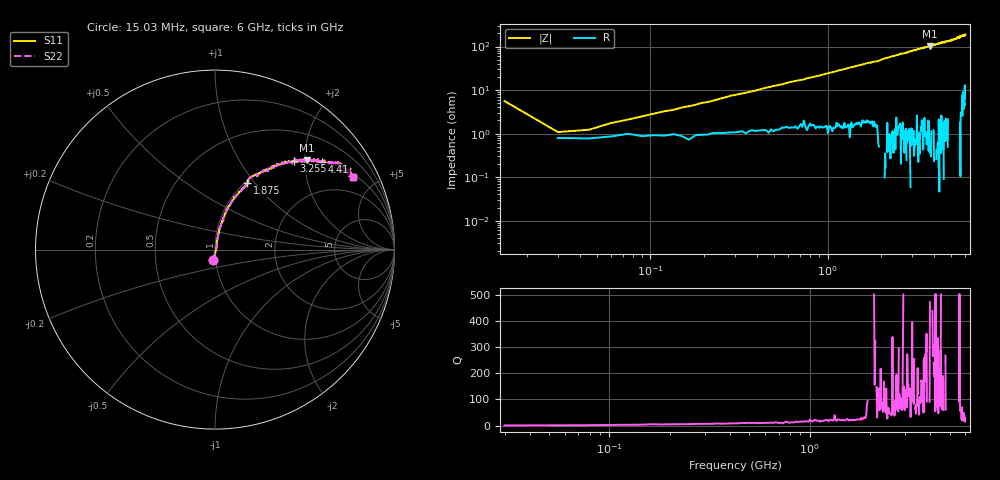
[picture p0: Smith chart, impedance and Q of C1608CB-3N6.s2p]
!	Network	Analyzer	HP8753E.07.74:	Oct	30	2002	Serial	No.	JP38451487
!	Hewlett-Packard
!	27	Aug	2009	15:19:33
!	Frequency	S11	S21	S12	S22
#	HZ	S	RI	R	50
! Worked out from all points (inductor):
!   400 points, 15.03 MHz to 6 GHz, reference 50 ohm
!   read as one part in series: L = 3.94 nH near 45.03 MHz
!   highest Q = 260 at 3.78 GHz (marker M1), where L = 4.32 nH
!   S11 on the Smith chart (normalised r, x): 15.03 MHz: 0.98, -0.11; 1.875 GHz: 1.03, +0.91; 3.255 GHz: 1.00, +1.77; 4.41 GHz: 1.01, +2.44; 6 GHz: 1.13, +3.73
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1.502992e7  -0.00853 -0.0557  1.01 0.0557  1.01 0.0557  -0.00853 -0.0557
3.002985e7  0.00785 0.00728  0.992 -0.00728  0.992 -0.00728  0.00785 0.00728
4.502978e7  0.00755 0.00938  0.992 -0.00938  0.992 -0.00938  0.00755 0.00938
6.00297e7  0.00855 0.015  0.991 -0.015  0.991 -0.015  0.00855 0.015
7.502962e7  0.0103 0.0182  0.99 -0.0182  0.99 -0.0182  0.0103 0.0182
1.200294e8  0.00975 0.0308  0.99 -0.0308  0.99 -0.0308  0.00975 0.0308
2.850286e8  0.0157 0.072  0.984 -0.072  0.984 -0.072  0.0157 0.072
6.150269e8  0.0354 0.145  0.965 -0.145  0.965 -0.145  0.0354 0.145
1.020025e9  0.0694 0.226  0.931 -0.226  0.931 -0.226  0.0694 0.226
1.875021e9  0.18 0.369  0.82 -0.369  0.82 -0.369  0.18 0.369
2.01002e9  0.198 0.401  0.802 -0.401  0.802 -0.401  0.198 0.401
3.015015e9  0.391 0.491  0.609 -0.491  0.609 -0.491  0.391 0.491
3.255014e9  0.439 0.495  0.561 -0.495  0.561 -0.495  0.439 0.495
3.780011e9  0.513 0.498  0.487 -0.498  0.487 -0.498  0.513 0.498
4.00501e9  0.551 0.504  0.449 -0.504  0.449 -0.504  0.551 0.504
4.410008e9  0.598 0.488  0.402 -0.488  0.402 -0.488  0.598 0.488
5.010005e9  0.665 0.481  0.335 -0.481  0.335 -0.481  0.665 0.481
5.355003e9  0.73 0.467  0.27 -0.467  0.27 -0.467  0.73 0.467
5.535002e9  0.706 0.437  0.294 -0.437  0.294 -0.437  0.706 0.437
5.565002e9  0.755 0.451  0.245 -0.451  0.245 -0.451  0.755 0.451
5.595002e9  0.721 0.443  0.279 -0.443  0.279 -0.443  0.721 0.443
6e9  0.769 0.404  0.231 -0.404  0.231 -0.404  0.769 0.404
